(* Logix 5000 DataType export POINT; software revision 30.00 *)

TYPE POINT :   // A point on an Edwards-curve represented in extended homogeneous coordinates
STRUCT
   X : DINT[22];
   Y : DINT[22];
   Z : DINT[22];
   T : DINT[22];
END_STRUCT
END_TYPE
